(* Logix 5000 AddOnInstructionDefinition export AMP_Configuration_Settings; software revision 20.04 *)

ADD_ON_INSTRUCTION AMP_Configuration_Settings   (* revision 1.0 *)
// Applied Motion - Configuration Settings AOI
// Help:
// The Configuration Settings AOI accepts all the required parameters for: Position Fault (PF), Control Mode (CM), Secondary Control Mode (CN), Electronic Gearing (EG), Input Noise Filter (EI), Jerk Filter (KJ), and then scales and issues these to the drive, one at a time.
VAR_IN_OUT
   MSG_Write : SINT[8]; {required}   // Message Write data tag
        [0]   // Message Reserved = 0
        [1]   // Message Type (16#01 or 16#02)
        [2]   // Type 1: Register Type 2: Opcode
        [3]   // Type 1: Opcode Type 2: Operand
        [4]   // Type 1: Parameter 1 Type 2: data MSB
        [5]   // Type 1: Parameter 2 Type 2: data LSB
        [6]   // Type 1: Parameter 3 Type 2: not used
        [7]   // Type 1: Parameter 4 Type 2: not used
   SendMsg : MESSAGE; {required}   // Message tag
   MSG_Response : SINT[8]; {required}   // Message Response data tag
        [0]   // Command Word
        [1]   // Jog Speed (0.25 rev/min)
        [2]   // Jog Acceleration (10 rev/s/s)
        [3]   // Jog Deceleration (10 rev/s/s)
        [4]   // Point-to-Point Velocity (0.25 rev/min)
        [5]   // Point-to-Point Acceleration (10 rev/s/s)
        [6]   // Point-to-Point Deceleration (10 rev/s/s)
        [7]   // Point-to-Point Distance (Motor steps)
        [9]   // (2x ASCII Letters in 16 lower word)
        [10]   // Data/Register 1
        [11]   // Data/Register 2
END_VAR
VAR_INPUT
   Configure : BOOL; {required}   // Start the Configuration
   PF : INT; {required}   // Position Fault (steps or counts)
   CM : INT; {required}   // Control Mode (integer code)
   CN : INT; {required}   // Secondary Control Mode (integer code)
   EG : INT; {required}   // Electronic Gearing (steps/rev or counts/rev)
   EI : INT; {required}   // Input Noise Filter Constant (0-255)
   KJ : INT; {required}   // Jerk Filter (Hz)
END_VAR
VAR_OUTPUT
   Sent : BOOL; {access Read Only, visible}   // All configuration settings have been sent to drive
   In_Progress : BOOL; {access Read Only, visible}   // The configuration is in progress
   Done : BOOL; {access Read Only, visible}   // Configuration completed without errors
   Error : BOOL; {access Read Only, visible}   // Configuration failed to complete - drive not ready or faulted
   State : DINT := 34; {access Read Only}   // Internal state of progress
END_VAR
VAR
   Loc_Start_ONS : BOOL; {access None}
   loc_Steps_per_Rev_div_by_2 : DINT;
END_VAR

ROUTINE Logic   (* ladder *)
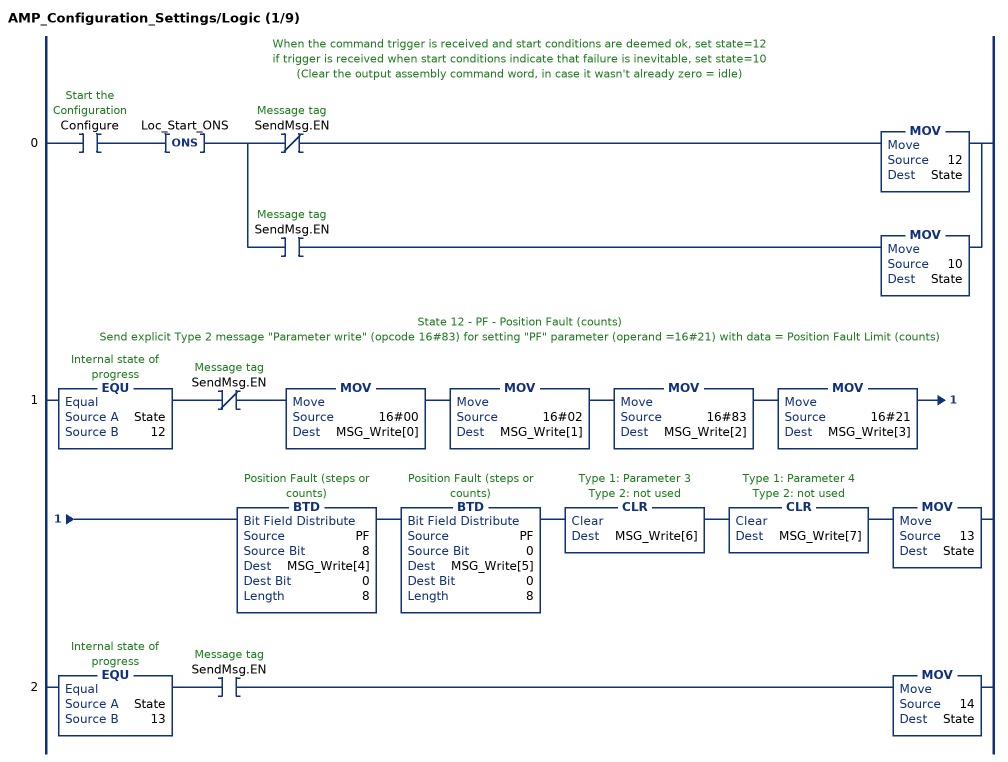
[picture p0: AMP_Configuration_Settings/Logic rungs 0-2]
   // When the command trigger is received and start conditions are deemed ok, set state=12
   // if trigger is received when start conditions indicate that failure is inevitable, set state=10
   // (Clear the output assembly command word, in case it wasn't already zero = idle)
   0: XIC(Configure)ONS(Loc_Start_ONS)[XIO(SendMsg.EN) MOV(12,State) ,XIC(SendMsg.EN) MOV(10,State) ];
   // State 12 - PF - Position Fault (counts)
   // Send explicit Type 2 message "Parameter write" (opcode 16#83) for setting "PF" parameter (operand =16#21) with data = Position Fault Limit (counts)
   1: EQU(State,12)XIO(SendMsg.EN)MOV(16#00,MSG_Write[0])MOV(16#02,MSG_Write[1])MOV(16#83,MSG_Write[2])MOV(16#21,MSG_Write[3])BTD(PF,8,MSG_Write[4],0,8)BTD(PF,0,MSG_Write[5],0,8)CLR(MSG_Write[6])CLR(MSG_Write[7])MOV(13,State);
   2: EQU(State,13)XIC(SendMsg.EN)MOV(14,State);
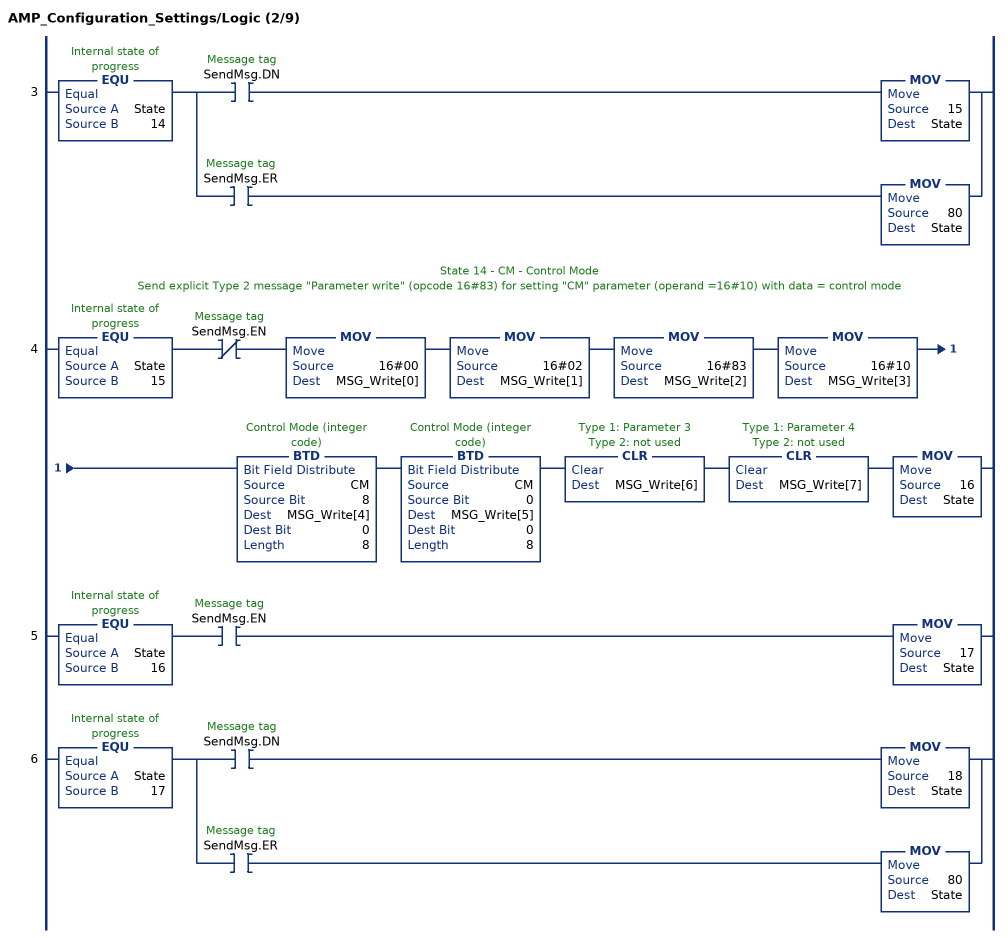
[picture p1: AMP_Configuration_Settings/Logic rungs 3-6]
   3: EQU(State,14)[XIC(SendMsg.DN) MOV(15,State) ,XIC(SendMsg.ER) MOV(80,State) ];
   // State 14 - CM - Control Mode
   // Send explicit Type 2 message "Parameter write" (opcode 16#83) for setting "CM" parameter (operand =16#10) with data = control mode
   4: EQU(State,15)XIO(SendMsg.EN)MOV(16#00,MSG_Write[0])MOV(16#02,MSG_Write[1])MOV(16#83,MSG_Write[2])MOV(16#10,MSG_Write[3])BTD(CM,8,MSG_Write[4],0,8)BTD(CM,0,MSG_Write[5],0,8)CLR(MSG_Write[6])CLR(MSG_Write[7])MOV(16,State);
   5: EQU(State,16)XIC(SendMsg.EN)MOV(17,State);
   6: EQU(State,17)[XIC(SendMsg.DN) MOV(18,State) ,XIC(SendMsg.ER) MOV(80,State) ];
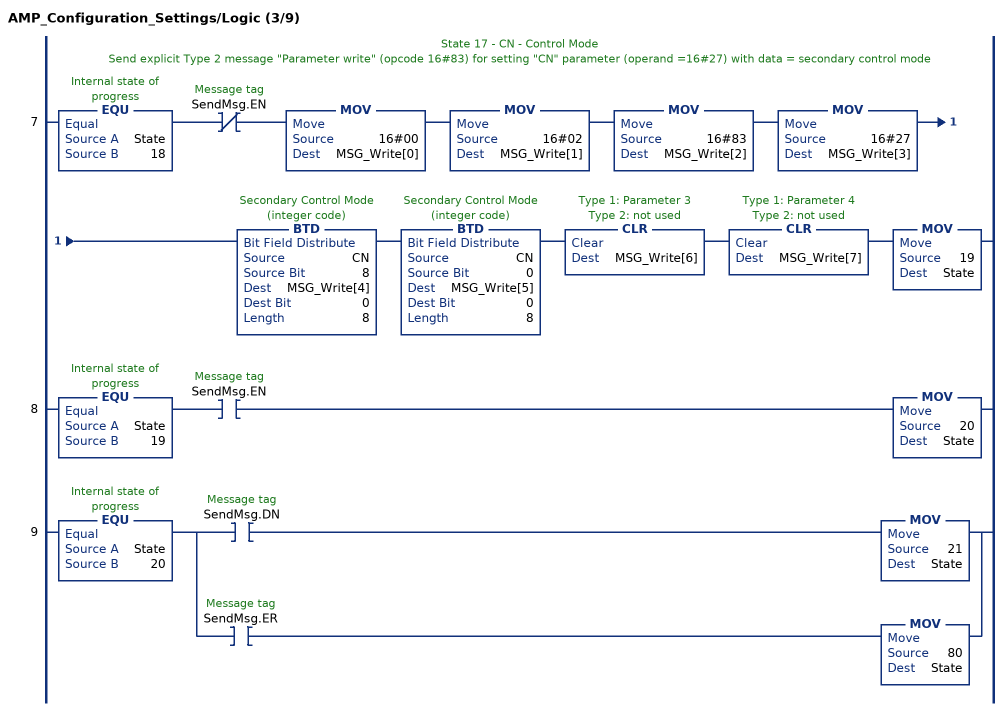
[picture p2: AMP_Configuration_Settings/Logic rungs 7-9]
   // State 17 - CN - Control Mode
   // Send explicit Type 2 message "Parameter write" (opcode 16#83) for setting "CN" parameter (operand =16#27) with data = secondary control mode
   7: EQU(State,18)XIO(SendMsg.EN)MOV(16#00,MSG_Write[0])MOV(16#02,MSG_Write[1])MOV(16#83,MSG_Write[2])MOV(16#27,MSG_Write[3])BTD(CN,8,MSG_Write[4],0,8)BTD(CN,0,MSG_Write[5],0,8)CLR(MSG_Write[6])CLR(MSG_Write[7])MOV(19,State);
   8: EQU(State,19)XIC(SendMsg.EN)MOV(20,State);
   9: EQU(State,20)[XIC(SendMsg.DN) MOV(21,State) ,XIC(SendMsg.ER) MOV(80,State) ];
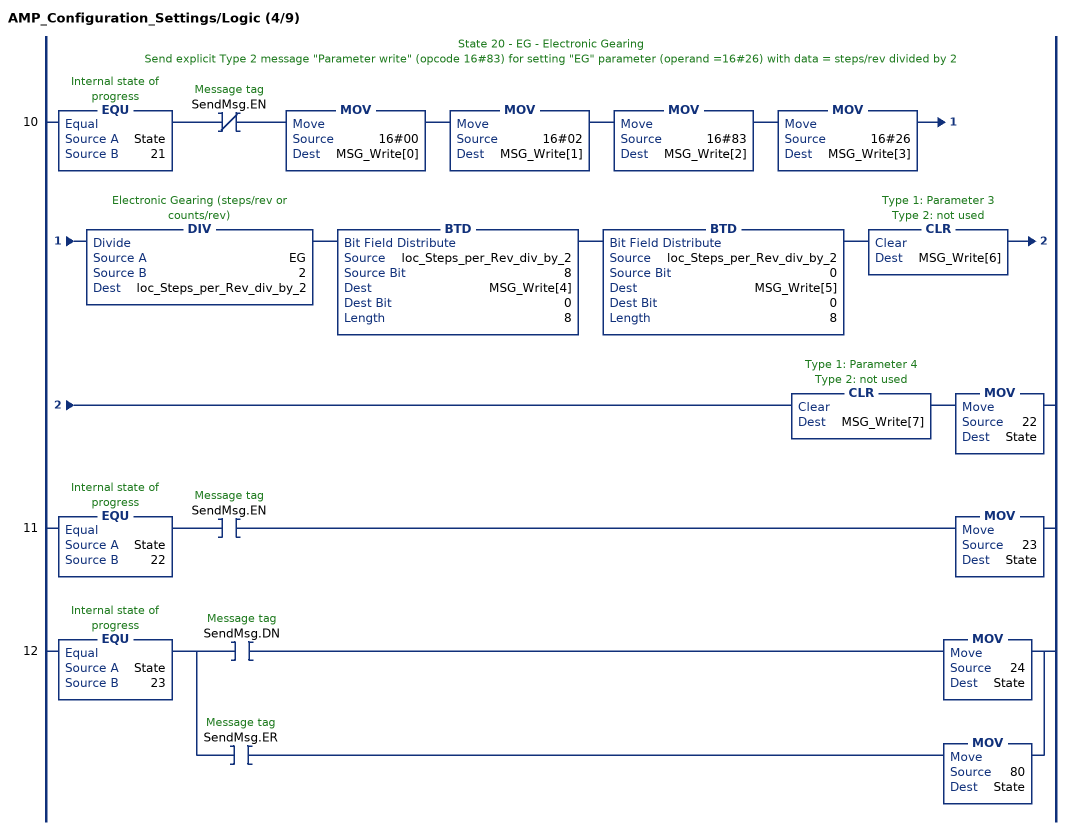
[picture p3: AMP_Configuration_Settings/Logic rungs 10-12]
   // State 20 - EG - Electronic Gearing
   // Send explicit Type 2 message "Parameter write" (opcode 16#83) for setting "EG" parameter (operand =16#26) with data = steps/rev divided by 2
   10: EQU(State,21)XIO(SendMsg.EN)MOV(16#00,MSG_Write[0])MOV(16#02,MSG_Write[1])MOV(16#83,MSG_Write[2])MOV(16#26,MSG_Write[3])DIV(EG,2,loc_Steps_per_Rev_div_by_2)BTD(loc_Steps_per_Rev_div_by_2,8,MSG_Write[4],0,8)BTD(loc_Steps_per_Rev_div_by_2,0,MSG_Write[5],0,8)CLR(MSG_Write[6])CLR(MSG_Write[7])MOV(22,State);
   11: EQU(State,22)XIC(SendMsg.EN)MOV(23,State);
   12: EQU(State,23)[XIC(SendMsg.DN) MOV(24,State) ,XIC(SendMsg.ER) MOV(80,State) ];
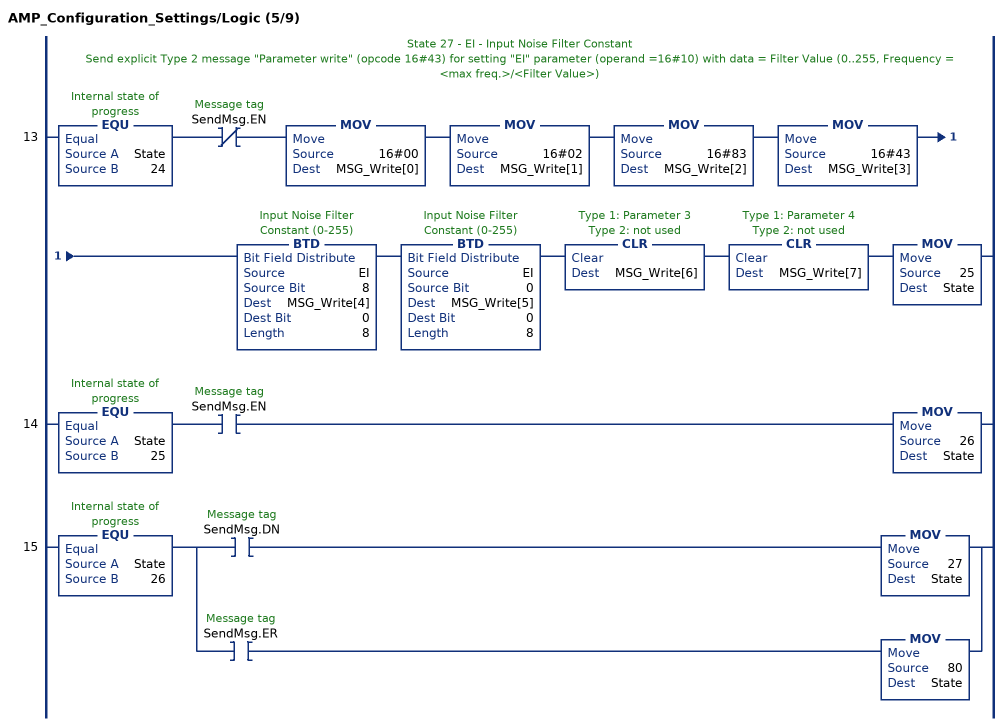
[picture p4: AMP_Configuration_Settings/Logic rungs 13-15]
   // State 27 - EI - Input Noise Filter Constant
   // Send explicit Type 2 message "Parameter write" (opcode 16#43) for setting "EI" parameter (operand =16#10) with data = Filter Value (0..255, Frequency = <max freq.>/<Filter Value>)
   13: EQU(State,24)XIO(SendMsg.EN)MOV(16#00,MSG_Write[0])MOV(16#02,MSG_Write[1])MOV(16#83,MSG_Write[2])MOV(16#43,MSG_Write[3])BTD(EI,8,MSG_Write[4],0,8)BTD(EI,0,MSG_Write[5],0,8)CLR(MSG_Write[6])CLR(MSG_Write[7])MOV(25,State);
   14: EQU(State,25)XIC(SendMsg.EN)MOV(26,State);
   15: EQU(State,26)[XIC(SendMsg.DN) MOV(27,State) ,XIC(SendMsg.ER) MOV(80,State) ];
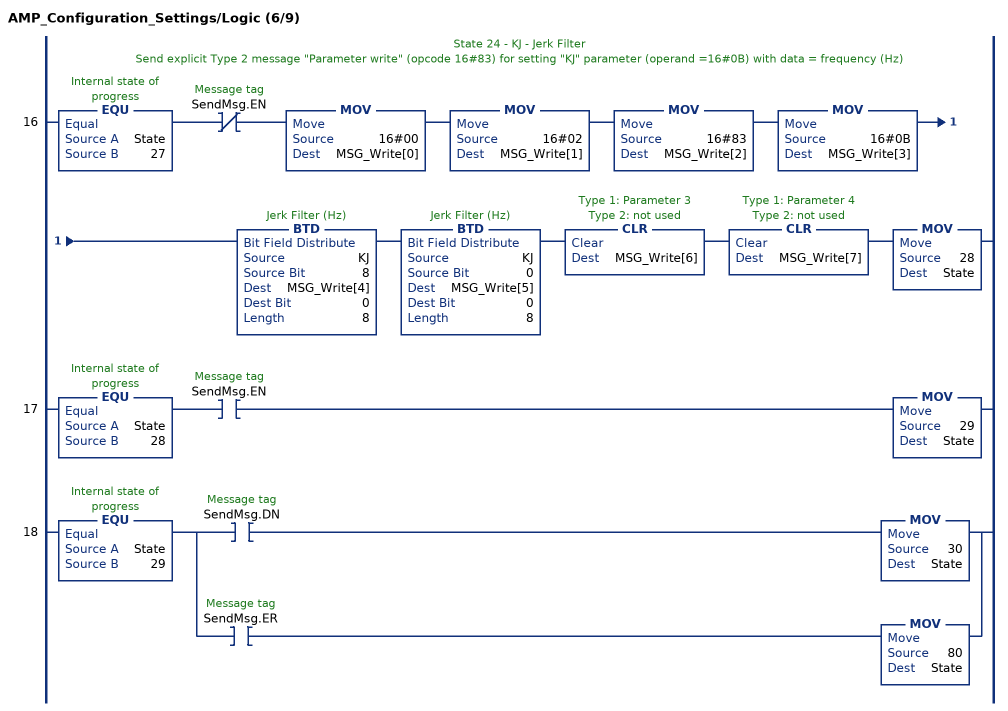
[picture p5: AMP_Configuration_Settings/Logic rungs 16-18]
   // State 24 - KJ - Jerk Filter
   // Send explicit Type 2 message "Parameter write" (opcode 16#83) for setting "KJ" parameter (operand =16#0B) with data = frequency (Hz)
   16: EQU(State,27)XIO(SendMsg.EN)MOV(16#00,MSG_Write[0])MOV(16#02,MSG_Write[1])MOV(16#83,MSG_Write[2])MOV(16#0B,MSG_Write[3])BTD(KJ,8,MSG_Write[4],0,8)BTD(KJ,0,MSG_Write[5],0,8)CLR(MSG_Write[6])CLR(MSG_Write[7])MOV(28,State);
   17: EQU(State,28)XIC(SendMsg.EN)MOV(29,State);
   18: EQU(State,29)[XIC(SendMsg.DN) MOV(30,State) ,XIC(SendMsg.ER) MOV(80,State) ];
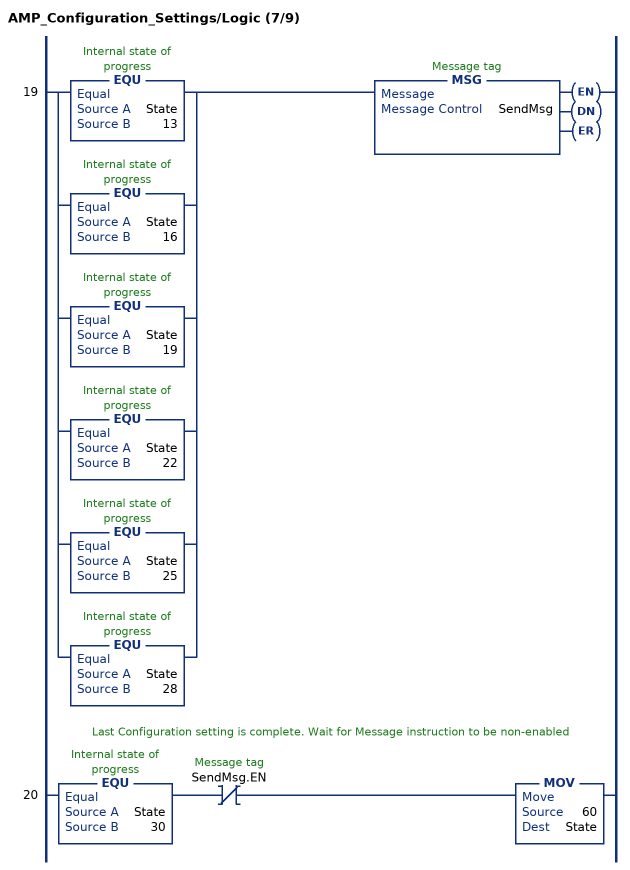
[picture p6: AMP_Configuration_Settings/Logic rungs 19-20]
   19: [EQU(State,13) ,EQU(State,16) ,EQU(State,19) ,EQU(State,22) ,EQU(State,25) ,EQU(State,28) ]MSG(SendMsg);
   // Last Configuration setting is complete. Wait for Message instruction to be non-enabled
   20: EQU(State,30)XIO(SendMsg.EN)MOV(60,State);
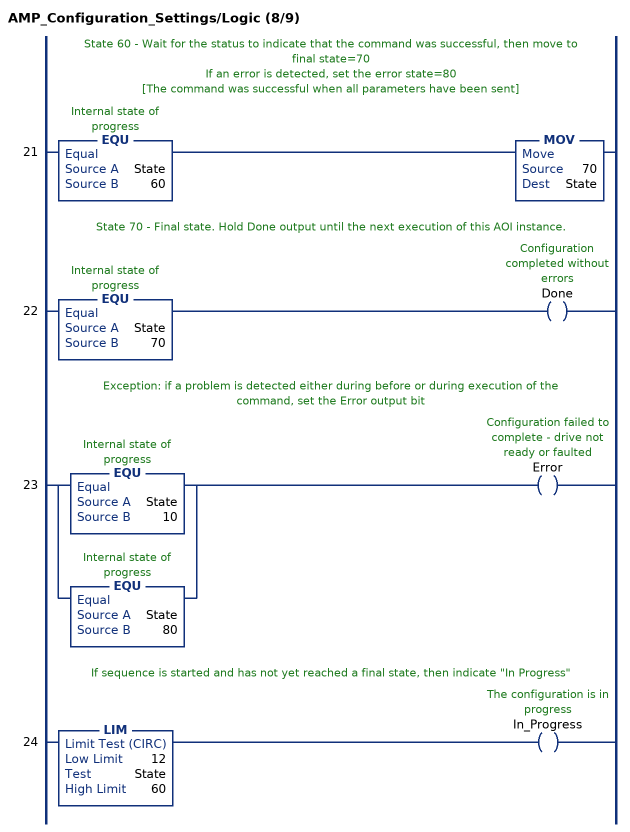
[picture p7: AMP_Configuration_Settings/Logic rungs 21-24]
   // State 60 - Wait for the status to indicate that the command was successful, then move to final state=70
   // If an error is detected, set the error state=80
   // [The command was successful when all parameters have been sent]
   21: EQU(State,60)MOV(70,State);
   // State 70 - Final state. Hold Done output until the next execution of this AOI instance.
   22: EQU(State,70)OTE(Done);
   // Exception: if a problem is detected either during before or during execution of the command, set the Error output bit
   23: [EQU(State,10) ,EQU(State,80) ]OTE(Error);
   // If sequence is started and has not yet reached a final state, then indicate "In Progress"
   24: LIM(12,State,60)OTE(In_Progress);
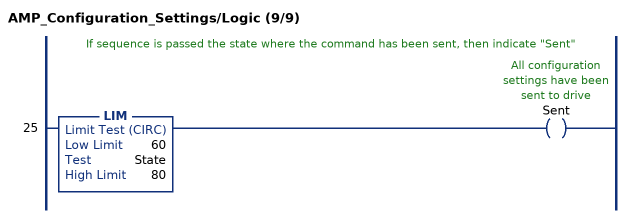
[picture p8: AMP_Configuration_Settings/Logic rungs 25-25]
   // If sequence is passed the state where the command has been sent, then indicate "Sent"
   25: LIM(60,State,80)OTE(Sent);
END_ROUTINE
END_ADD_ON_INSTRUCTION
